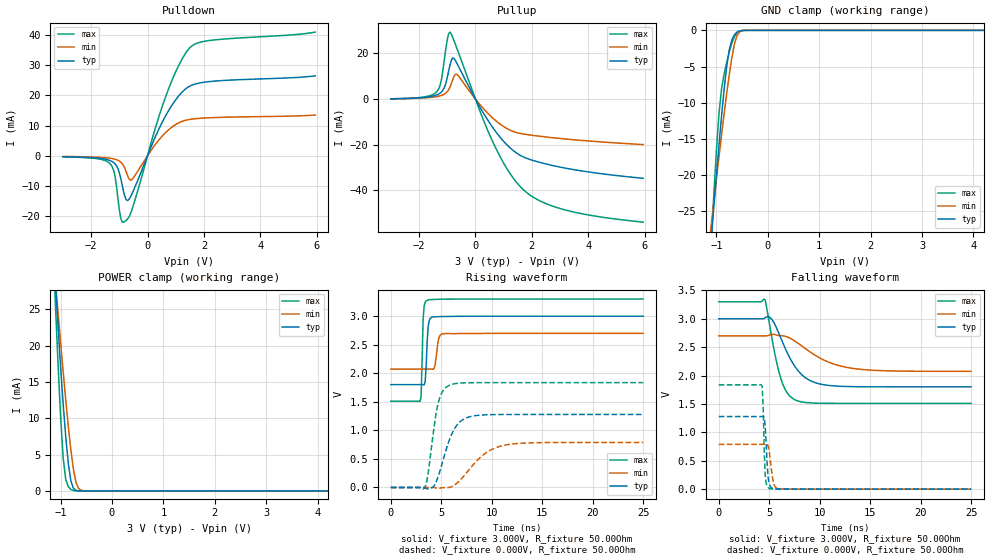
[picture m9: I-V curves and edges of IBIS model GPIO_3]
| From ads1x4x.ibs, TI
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|   GPIO 3.0V Model
[Model]   GPIO_3
Model_type   I/O
|Signals   REFP0_GPIO0 REFN0_GPIO1 AIN4_IEXC_GPIO4 AIN5_IEXC_GPIO5
|AIN6_IEXC_GPIO6 AIN7_IEXC_GPIO7 AIN2_IEXC_GPIO2 AIN3_IEXC_GPIO3
Vinl =  0.75V
Vinh =  2.00V
| variable   typ   min   max
|C_comp Output Disabled
C_comp   1.803pF   2.171pF   1.527pF
|C_comp Output Low
|C_comp   5.409pF   5.953pF   4.554pF
|C_comp Output High
|C_comp   4.749pF   5.542pF   4.605pF
[Model Spec]
|Timing spec test load voltage corners 0.45*VCC
Vmeas   2.5V   2.375V   2.625V
Vref   2.5V   2.375V   2.625V
|Junction Temperature
[Temperature Range]   40.0   105.0   -40.0
[Voltage range]   5.0V   4.75V   5.25V
[Pullup reference]   3.0V   2.7V   3.3V
[power clamp reference]   3.0V   2.7V   3.3V
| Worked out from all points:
|   slope of the pulldown table from 0 to 0.45 V, typ, clamps not added: 46.2 ohm
|   slope of the pullup table from 0 to 0.45 V, typ, clamps not added: 47.4 ohm
|   GND clamp passes 1 mA (typ) near -0.68 V on its own axis
|   POWER clamp passes 1 mA (typ) near -0.78 V on its own axis
|   falling waveform, V_fixture 3.000V, R_fixture 50.00Ohm: 20-80 % time 2.17ns typ, 3.65ns min, 1.31ns max; typ from 3 V to 1.8 V
|   rising waveform, V_fixture 3.000V, R_fixture 50.00Ohm: 20-80 % time 207ps typ, 274ps min, 156ps max; typ from 1.8 V to 3 V
|   rising waveform, V_fixture 0.000V, R_fixture 50.00Ohm: 20-80 % time 1.48ns typ, 2.62ns min, 897ps max; typ from 0 V to 1.28 V
|   falling waveform, V_fixture 0.000V, R_fixture 50.00Ohm: 20-80 % time 245ps typ, 347ps min, 178ps max; typ from 1.28 V to 0 V
[Pulldown]
|   Voltage   I(typ)   I(min)   I(max)
-3V       -312uA     -207.5uA   -348.3uA
-1.3V     -1.685mA   -831.9uA   -2.891mA
-1.15V    -2.673mA   -1.125mA   -6.794mA
-1.05V    -4.187mA   -1.463mA   -13.94mA
-950mV    -7.395mA   -2.055mA   -20.58mA
-850mV    -11.76mA   -3.233mA   -21.92mA
-700mV    -14.73mA   -6.717mA   -20.78mA
-550mV    -12.57mA   -7.815mA   -17.77mA
600mV     12.48mA    7.274mA    18.37mA
1.1V      19.7mA     10.86mA    29.71mA
1.5V      23.02mA    12.02mA    35.68mA
5.95V     26.4mA     13.46mA    40.86mA
[GND Clamp]
|   Voltage   I(typ)   I(min)   I(max)
-3V       -210mA     -153.4mA   -322.5mA
-1.1V     -28.82mA   -26.84mA   -29.34mA
-1.05V    -24.39mA   -23.68mA   -22.68mA
-1V       -20.05mA   -20.56mA   -16.59mA
-950mV    -15.85mA   -17.49mA   -11.52mA
-900mV    -11.85mA   -14.48mA   -8.111mA
-800mV    -5.026mA   -8.749mA   -4.411mA
-750mV    -2.711mA   -6.126mA   -2.987mA
-650mV    -613.9uA   -1.925mA   -868.3uA
-600mV    -244.8uA   -736.3uA   -329.6uA
-550mV    -83.37uA   -214.1uA   -95.6uA
5.95V     0A         0A         0A
[Pullup]
|   Voltage   I(typ)   I(min)   I(max)
-3V       92.55uA    87.73uA    78.42uA
-1.35V    1.911mA    1.115mA    3.516mA
-1.2V     3.156mA    1.593mA    8.875mA
-1.1V     5.097mA    2.157mA    17.52mA
-1V       9.366mA    3.19mA     25.97mA
-900mV    15.01mA    5.304mA    29.4mA
-800mV    18.06mA    8.717mA    26.9mA
-650mV    15.5mA     10.79mA    22.01mA
650mV     -13.15mA   -8.755mA   -19.72mA
1.65V     -25.15mA   -15.28mA   -39.27mA
3.1V      -30.17mA   -17.46mA   -48.47mA
5.95V     -34.86mA   -20.03mA   -54.13mA
[POWER Clamp]
|   Voltage   I(typ)   I(min)   I(max)
-3V       210.3mA    181mA      249.3mA
-1.15V    35.1mA     33.46mA    34.21mA
-1.1V     28.8mA     28.98mA    25.73mA
-1.05V    22.77mA    24.68mA    17.65mA
-1V       17.16mA    20.52mA    10.34mA
-950mV    12.05mA    16.49mA    4.629mA
-900mV    7.526mA    12.61mA    1.596mA
-850mV    3.817mA    8.951mA    598.2uA
-750mV    368.1uA    2.965mA    48.18uA
-650mV    17.55uA    343.9uA    1.801uA
-550mV    887.2nA    19.64uA    56.62nA
5.95V     0A         0A         0A
[Ramp]
R_load = 50.00Ohm
|   typ   min   max
dV/dt_r   767.134mV/1.482ns   473.243mV/2.625ns   1.102V/897.087ps
dV/dt_f   719.061mV/2.168ns   375.411mV/3.652ns   1.073V/1.314ns
[Falling Waveform]
V_fixture = 3.000V
V_fixture_min = 2.700V
V_fixture_max = 3.300V
R_fixture = 50.00Ohm
|   Time   V(typ)   V(min)   V(max)
0s        3V         2.7V       3.3V
4.6ns     3.02V      2.7V       3.333V
5.3ns     2.98V      2.724V     2.627V
5.7ns     2.847V     2.714V     2.263V
6.1ns     2.682V     2.703V     1.98V
6.8ns     2.398V     2.68V      1.692V
7.7ns     2.122V     2.588V     1.562V
9.5ns     1.879V     2.364V     1.516V
12.9ns    1.807V     2.137V     1.511V
25ns      1.802V     2.074V     1.511V
[Rising Waveform]
V_fixture = 3.000V
V_fixture_min = 2.700V
V_fixture_max = 3.300V
R_fixture = 50.00Ohm
|   Time   V(typ)   V(min)   V(max)
0s        1.802V     2.074V     1.511V
2.9ns     1.802V     2.074V     1.508V
3ns       1.801V     2.074V     1.596V
3.2ns     1.8V       2.074V     2.951V
3.4ns     1.851V     2.074V     3.243V
3.6ns     2.559V     2.074V     3.279V
3.9ns     2.96V      2.074V     3.29V
4.3ns     2.988V     2.091V     3.294V
5.2ns     2.994V     2.692V     3.298V
25ns      3V         2.7V       3.3V
[Rising Waveform]
V_fixture = 0.000V
V_fixture_min = 0.000V
V_fixture_max = 0.000V
R_fixture = 50.00Ohm
|   Time   V(typ)   V(min)   V(max)
0s        1.322nV    1.591nV    1.191nV
3.4ns     -6.205mV   2.457uV    5.689mV
3.7ns     -22.52mV   37.61uV    256.5mV
4.2ns     10.63mV    -35.66uV   946.1mV
4.7ns     195.1mV    -18.85mV   1.481V
5.8ns     831.4mV    2.301mV    1.79V
7.4ns     1.213V     235.6mV    1.833V
9.3ns     1.272V     589.9mV    1.836V
11.2ns    1.278V     737.3mV    1.836V
25ns      1.279V     788.7mV    1.836V
[Falling Waveform]
V_fixture = 0.000V
V_fixture_min = 0.000V
V_fixture_max = 0.000V
R_fixture = 50.00Ohm
|   Time   V(typ)   V(min)   V(max)
0s        1.279V     788.7mV    1.836V
4.3ns     1.281V     788.6mV    1.809V
4.4ns     1.284V     789mV      1.463V
4.5ns     1.267V     789.9mV    726.8mV
4.6ns     1.12V      791.7mV    252.7mV
4.8ns     436.1mV    790.9mV    52.39mV
5ns       92.63mV    667.1mV    12.87mV
5.4ns     11mV       129.4mV    2.985mV
5.9ns     3.125mV    10.91mV    1.758mV
25ns      1.322nV    1.591nV    1.191nV
